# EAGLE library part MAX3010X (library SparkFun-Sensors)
MAX30105 High Sensitivity Optical Sensor Can be used for Pulse Detection, Pulse Ox, and possible visual particle detection. I2C communication. Datasheet SparkFun Products: SparkFun Particle Sensor Breakout - MAX30105
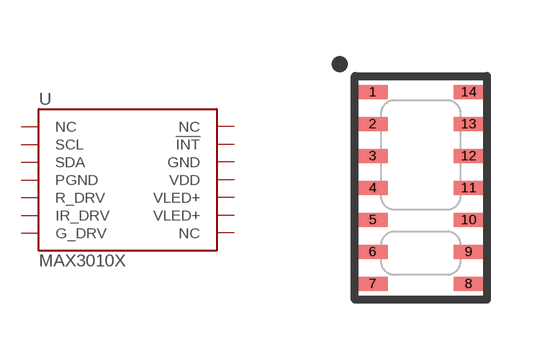
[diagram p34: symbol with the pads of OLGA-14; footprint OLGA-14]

Designator prefix U

## MAX3010X-30105 (PROD_ID: IC-13510; VALUE: MAX30105)  [OLGA-14]
1  NC
2  SCL
3  SDA
4  PGND
5  R_DRV
6  IR_DRV
7  G_DRV
8  NC
9  VLED+
10  VLED+
11  VDD
12  GND
13  !INT
14  NC

## MAX3010X-30102 (PROD_ID: IC-14316; VALUE: 30102)  [OLGA-14]
Pads as for OLGA-14

## Footprint OLGA-14 (pad centres in mm)
OLGA - 14 Pin Specifications: Pin count: 14 Datasheet referenced for footprint Example device(s): MAX30105
smd 0.75 x 0.35: 1 -1.2,2.4; 2 -1.2,1.6; 3 -1.2,0.8; 4 -1.2,0; 5 -1.2,-0.8; 6 -1.2,-1.6; 7 -1.2,-2.4; 8 1.2,-2.4; 9 1.2,-1.6; 10 1.2,-0.8; 11 1.2,0; 12 1.2,0.8; 13 1.2,1.6; 14 1.2,2.4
